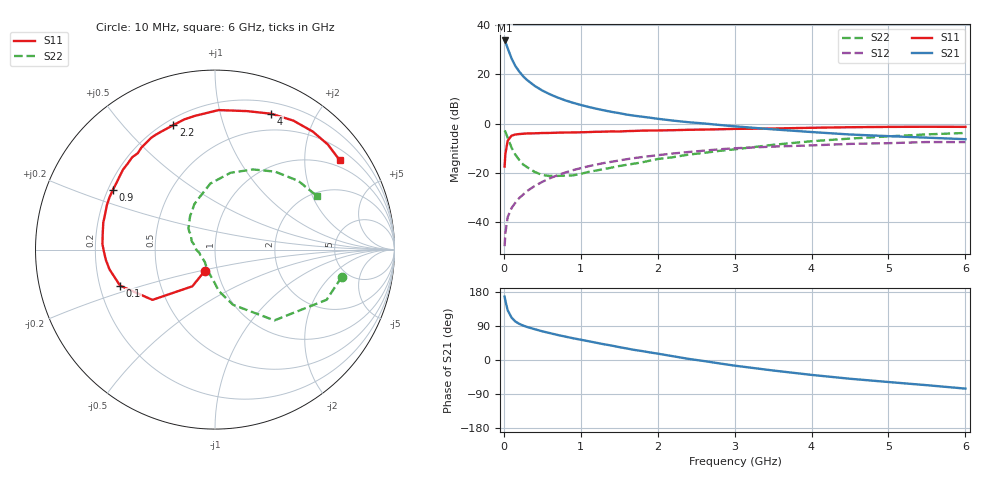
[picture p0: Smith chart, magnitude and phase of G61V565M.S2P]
! SIEMENS Small Signal Semiconductors
! BFG193
! Si NPN RF Bipolar Junction Transistor in SOT223
! VCE = 1.5 V  IC = 65 mA
! Common Emitter S-Parameters:  August  1996
# GHz  S  MA  R  50
!  f  S11  S21  S12  S22
! GHz  MAG  ANG  MAG  ANG  MAG  ANG  MAG  ANG
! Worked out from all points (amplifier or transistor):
!   36 points, 10 MHz to 6 GHz, reference 50 ohm
!   highest |S21| = 33.8 dB at 10 MHz (marker M1)
!   |S21| within 3 dB of that: start of sweep to 47.89 MHz
!   unconditionally stable (mu >= 1): start of sweep to 17.57 MHz; 199.1 MHz to 4.334 GHz; 5.671 GHz to end of sweep
!   at 250 MHz: K = 1.06, MAG = 22.6 dB, |S12| = -28.9 dB
!   at 1.4 GHz: K = 1.11, MAG = 8.1 dB, |S12| = -15.6 dB
!   at 6 GHz: K = 1.02, MAG = -0.2 dB, |S12| = -7.6 dB
!   S11 on the Smith chart (normalised r, x): 10 MHz: 0.87, -0.21; 100 MHz: 0.29, -0.17; 900 MHz: 0.22, +0.26; 2.2 GHz: 0.23, +0.69; 4 GHz: 0.31, +1.45; 6 GHz: 0.79, +2.93
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0.01  0.1336 -115.7  48.95 167.3  0.0032 76.8  0.7225 -12.1
0.02  0.2404 -121.7  45.79 156.2  0.0059 71.6  0.6819 -24.2
0.05  0.447 -141.2  33.93 131.2  0.0125 62.4  0.5148 -50.0
0.1  0.5658 -159.2  21.16 112.0  0.0191 61.2  0.3234 -71.9
0.15  0.5981 -169.4  14.78 101.5  0.0245 62.2  0.2323 -84.7
0.2  0.6105 -174.5  11.42 95.5  0.0305 65.2  0.1817 -91.3
0.25  0.6195 -179.2  9.179 90.9  0.0357 66.1  0.1473 -99.7
0.3  0.6279 177.2  7.721 87.3  0.0421 67.1  0.1301 -105.8
0.4  0.6321 171.7  5.843 81.4  0.0535 67.9  0.1038 -118.5
0.5  0.6405 166.4  4.686 75.7  0.0652 66.3  0.0896 -129.1
0.6  0.6438 161.8  3.925 70.9  0.0772 65.5  0.0858 -138.6
0.7  0.6514 157.6  3.373 66.0  0.0891 64.0  0.0861 -149.0
0.9  0.6592 149.8  2.639 57.4  0.1127 59.9  0.0882 -167.4
1.1  0.6697 142.6  2.176 49.6  0.1351 56.0  0.1037 -179.2
1.6  0.7005 125.9  1.517 30.3  0.1883 44.2  0.145 155.7
2.2  0.7314 108.5  1.146 9.9  0.2459 29.6  0.2065 134.2
2.8  0.7637 93.0  0.936 -8.9  0.2988 14.9  0.2776 114.6
3.5  0.7921 76.9  0.761 -27.7  0.3395 -3.2  0.3689 94.0
4  0.8193 67.5  0.671 -39.3  0.3591 -13.0  0.4366 78.6
4.5  0.8409 58.7  0.598 -49.5  0.3853 -23.2  0.4938 64.7
5.5  0.8591 43.0  0.516 -66.5  0.4198 -46.1  0.6014 39.6
6  0.8549 35.5  0.48 -75.5  0.4191 -59.1  0.6425 27.6
